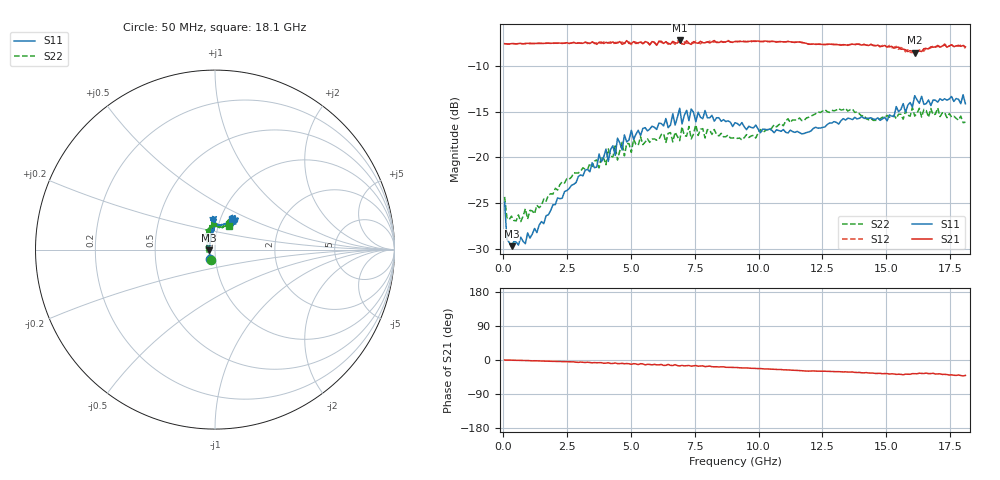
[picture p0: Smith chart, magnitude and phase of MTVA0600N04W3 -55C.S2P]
! Network Analyzer HP8720D.06.14 Serial No. US36140669
!  8 Jul 2005  11:33:58
! Frequency  S11  S21  S12  S22
# HZ  S  DB R 50
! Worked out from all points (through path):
!   201 points, 50 MHz to 18.1 GHz, reference 50 ohm
!   highest |S21| = -7.27 dB at 6.909 GHz (marker M1); lowest = -8.6 dB at 16.11 GHz (marker M2)
!   group delay of S21, straight-line fit = 6.61 ps
!   lowest |S11| = -29.7 dB at 320.8 MHz (marker M3), VSWR 1.07, Z = 46.8 - j0.354 ohm
!   |S11| at or under -10 dB: start of sweep to end of sweep
!   |S22| runs from -27.0 to -14.6 dB; largest |S21 - S12| = 0.018
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5e7  -24.88 -118.9  -7.61 -0.0  -7.62 -0.1  -24.29 -110.7
1.4025e8  -28.91 -148.0  -7.65 -0.3  -7.63 -0.1  -26.56 -154.2
3.2075e8  -29.66 -173.4  -7.61 -0.5  -7.63 -0.4  -26.39 -174.9
9.525e8  -28.23 150.8  -7.58 -1.4  -7.61 -1.4  -26.71 158.2
3.1185e9  -22.00 106.9  -7.57 -5.9  -7.59 -6.3  -21.14 122.2
4.021e9  -19.09 100.8  -7.47 -8.2  -7.58 -7.5  -20.80 113.8
4.382e9  -19.78 96.9  -7.58 -7.8  -7.49 -9.3  -18.75 113.3
4.47225e9  -17.91 92.3  -7.53 -9.5  -7.48 -8.2  -20.28 116.2
4.65275e9  -19.18 92.1  -7.68 -8.8  -7.43 -9.6  -18.35 114.7
4.743e9  -17.55 95.5  -7.57 -9.9  -7.59 -9.0  -19.84 110.5
5.104e9  -18.04 97.7  -7.39 -9.6  -7.41 -10.8  -18.02 106.1
6.09675e9  -16.26 92.8  -7.38 -12.8  -7.33 -12.7  -18.03 102.2
6.7285e9  -16.48 97.0  -7.50 -12.3  -7.69 -13.7  -17.25 95.9
6.909e9  -14.65 94.2  -7.27 -15.7  -7.46 -14.4  -18.17 93.3
6.99925e9  -16.35 93.7  -7.63 -14.2  -7.66 -16.0  -16.66 94.5
7.36025e9  -14.73 87.7  -7.70 -16.3  -7.51 -15.0  -17.98 98.3
7.54075e9  -16.12 89.1  -7.53 -14.6  -7.34 -16.7  -16.45 97.2
9.075e9  -16.23 95.0  -7.38 -19.7  -7.35 -19.8  -17.86 82.8
1.21435e10  -16.84 75.0  -7.65 -28.8  -7.61 -29.0  -15.38 66.6
1.512175e10  -15.37 53.7  -7.96 -37.1  -7.81 -36.7  -15.62 62.4
1.61145e10  -13.28 53.4  -8.59 -36.2  -8.31 -36.0  -15.49 61.6
1.81e10  -14.15 62.0  -7.97 -40.7  -8.13 -41.5  -16.16 59.0
